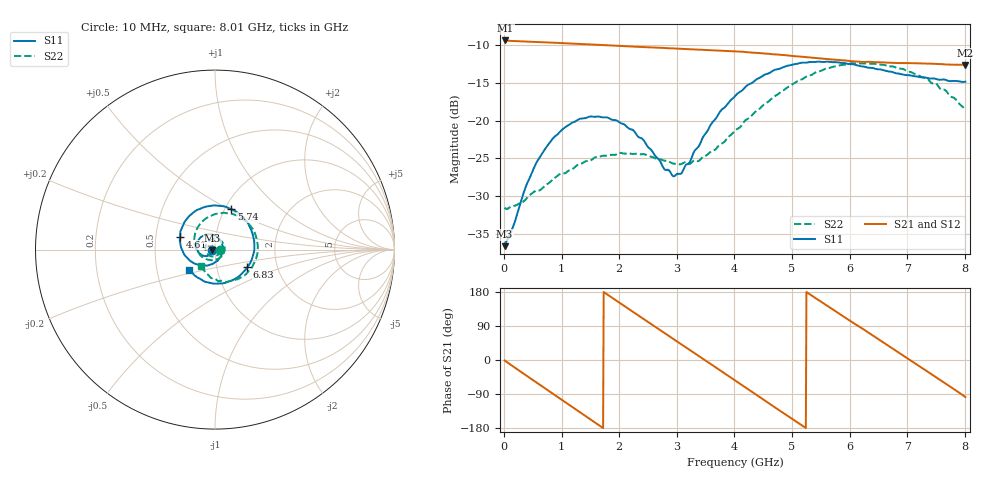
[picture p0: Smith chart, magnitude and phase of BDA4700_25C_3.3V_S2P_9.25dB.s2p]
!Agilent Technologies,E5071B,MY42404982,A.09.10
!Date: Mon Oct 20 18:06:53 2025
!Data & Calibration Information:
!Freq	S11:SOLT2(ON)	S21:SOLT2(ON)	S12:SOLT2(ON)	S22:SOLT2(ON)
# Hz S RI R 50
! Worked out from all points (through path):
!   801 points, 10 MHz to 8.01 GHz, reference 50 ohm
!   highest |S21| = -9.37 dB at 20 MHz (marker M1); lowest = -12.6 dB at 8.01 GHz (marker M2)
!   group delay of S21, straight-line fit = 283 ps
!   lowest |S11| = -36.6 dB at 10 MHz (marker M3), VSWR 1.03, Z = 48.6 - j0.139 ohm
!   |S11| at or under -10 dB: start of sweep to end of sweep
!   |S22| runs from -31.7 to -12.4 dB; largest |S21 - S12| = 0.0038
!   S11 on the Smith chart (normalised r, x): 10 MHz: 0.97, -0.00; 4.61 GHz: 0.67, +0.10; 5.74 GHz: 1.07, +0.52; 6.83 GHz: 1.40, -0.29; 8.01 GHz: 0.73, -0.17
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1e7  -0.0147 -0.00143  0.3398 -0.00724  0.3399 -0.00767  0.0265 -0.00135
2e7  -0.0152 -0.00225  0.3397 -0.0133  0.3396 -0.0143  0.0263 -0.00148
4.1e8  -0.0272 -0.028  0.2423 -0.23  0.2421 -0.2301  0.0194 -0.0243
7.2e8  -0.0547 -0.0361  0.0802 -0.3203  0.0803 -0.3202  -0.000899 -0.0373
1.02e9  -0.0852 -0.0226  -0.0962 -0.3119  -0.0961 -0.312  -0.0284 -0.0345
1.35e9  -0.1026 0.0139  -0.2517 -0.201  -0.2516 -0.2012  -0.0517 -0.00633
1.93e9  -0.0611 0.0803  -0.2926 0.1139  -0.2926 0.114  -0.0255 0.0536
2.32e9  -0.00439 0.0788  -0.1486 0.2705  -0.1485 0.2706  0.0218 0.0563
2.68e9  0.0365 0.042  0.0424 0.3013  0.0419 0.3012  0.0514 0.0214
2.93e9  0.043 0.00154  0.1662 0.2513  0.1659 0.2507  0.0511 -0.00979
3.07e9  0.0386 -0.0224  0.2226 0.2006  0.2205 0.2022  0.0438 -0.0272
3.53e9  -0.022 -0.0824  0.293 -0.0238  0.2932 -0.0243  -0.00844 -0.0589
4.01e9  -0.1276 -0.0696  0.17 -0.2326  0.1703 -0.2321  -0.0782 -0.0352
4.61e9  -0.1942 0.0726  -0.1189 -0.2501  -0.1183 -0.2505  -0.113 0.0756
5e9  -0.1468 0.1832  -0.2435 -0.113  -0.2441 -0.1138  -0.0666 0.1603
5.35e9  -0.0451 0.2404  -0.2568 0.0487  -0.2572 0.0472  0.0227 0.2007
5.74e9  0.0906 0.2265  -0.1636 0.1937  -0.1635 0.1936  0.14 0.1808
6.18e9  0.1976 0.1177  0.0141 0.2451  0.0166 0.2457  0.2289 0.0708
6.68e9  0.2052 -0.0534  0.1937 0.1454  0.1942 0.1451  0.2142 -0.0822
6.83e9  0.18 -0.099  0.2234 0.0904  0.2238 0.0891  0.1877 -0.1187
7.33e9  0.0435 -0.1877  0.2103 -0.1133  0.2105 -0.1137  0.0622 -0.1805
8.01e9  -0.1434 -0.1109  -0.0309 -0.2319  -0.0302 -0.2321  -0.0776 -0.0894
